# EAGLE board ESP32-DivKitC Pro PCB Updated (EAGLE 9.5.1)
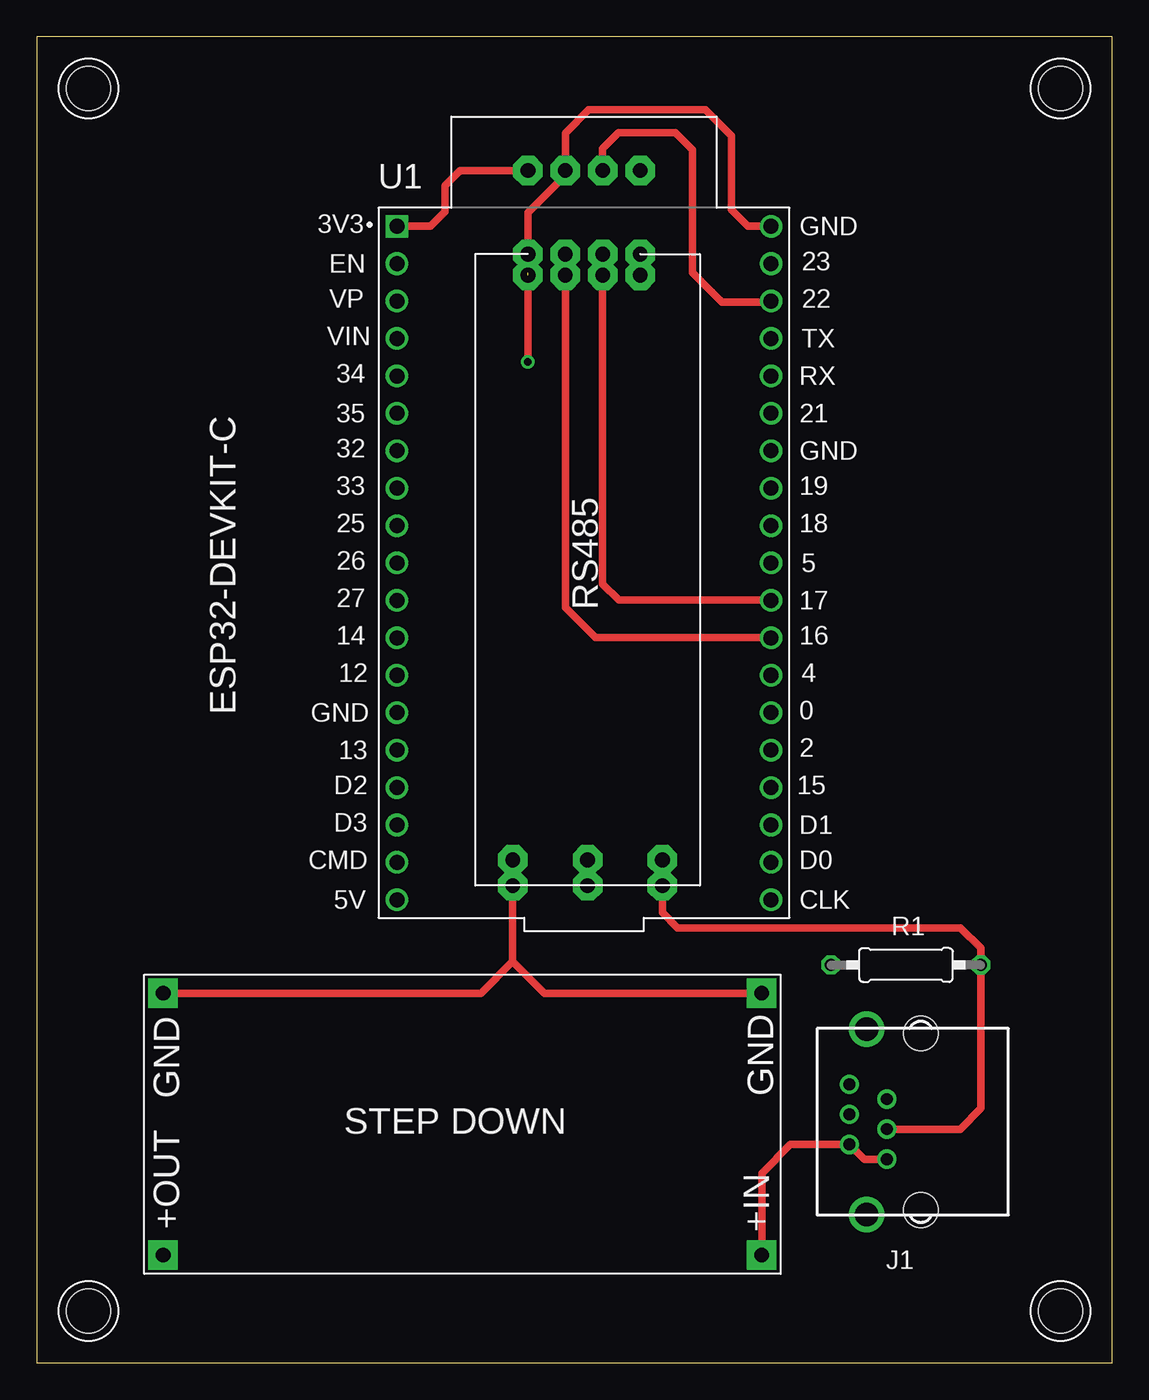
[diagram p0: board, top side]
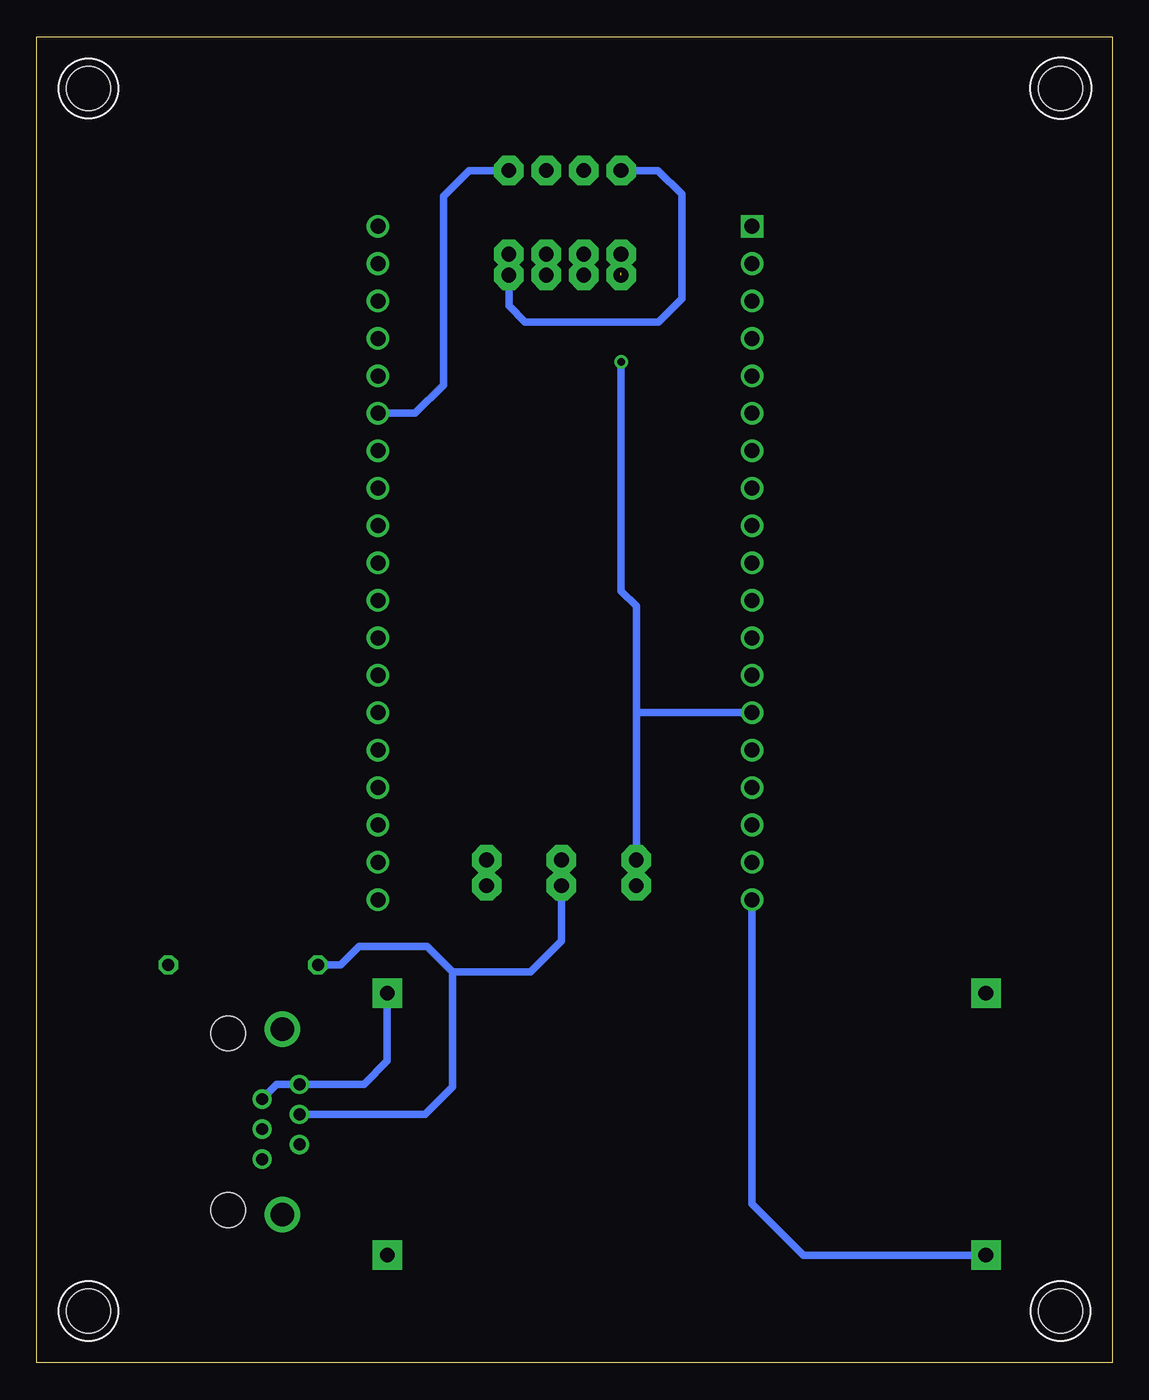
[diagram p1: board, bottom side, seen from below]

Size 73 x 90 mm. Coordinates in mm from the lower left corner, seen from the top.
Outline: 0,0 73,0 73,90 0,90 0,0
Copper layers (1*16): Top 0.035mm / dielectric 1.5mm / Bottom 0.035mm
Design rules "default *": minimum track width 6mil, minimum drill 0.2mm, track to track 6mil, track to pad 6mil, pad to pad 6mil, via to via 6mil, smd to smd 6mil, copper to edge 40mil, drill to drill 6mil, minimum pad ring 10mil, minimum via ring 8mil, stop-mask expansion 4mil, vias tented up to drill 0mil, thermal gap 10mil
Holes 3 mm at 3.5,3.5 3.5,86.5 69.5,86.5 69.5,3.5

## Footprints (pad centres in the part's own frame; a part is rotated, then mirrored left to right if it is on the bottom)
YH-55-10 = drill 0.8 pad 1.3: 1 -2.54,2.3; 2 -1.54,4.84; 3 -0.5,2.3; 4 0.5,4.84; 5 1.54,2.3; 6 2.54,4.84 | drill 1.6 pad 2.184: S1 -6.3,3.68; S2 6.3,3.68 | hole 2.36: -6,0; 6,0
0207/10 = drill 0.813 octagon: 1 -5.08,0; 2 5.08,0
MODULE_ESP32-DEVKITC = drill 1.02 square: 1 -12.7,22.85 | drill 1.02: 2 -12.7,20.31; 3 -12.7,17.77; 4 -12.7,15.23; 5 -12.7,12.69; 6 -12.7,10.15; 7 -12.7,7.61; 8 -12.7,5.07; 9 -12.7,2.53; 10 -12.7,-0.01; 11 -12.7,-2.55; 12 -12.7,-5.09; 13 -12.7,-7.63; 14 -12.7,-10.17; 15 -12.7,-12.71; 16 -12.7,-15.25; 17 -12.7,-17.79; 18 -12.7,-20.33; 19 -12.7,-22.87; 20 12.7,-22.87; 21 12.7,-20.33; 22 12.7,-17.79; 23 12.7,-15.25; 24 12.7,-12.71; 25 12.7,-10.17; 26 12.7,-7.63; 27 12.7,-5.09; 28 12.7,-2.55; 29 12.7,-0.01; 30 12.7,2.53; 31 12.7,5.07; 32 12.7,7.61; 33 12.7,10.15; 34 12.7,12.69; 35 12.7,15.23; 36 12.7,17.77; 37 12.7,20.31; 38 12.7,22.85

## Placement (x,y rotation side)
J1  RJ11  [YH-55-10]  60.01,16.35 90 top
R1  120R  [0207/10]  59,27 0 top
U1  ESP32-DEVKITC  [MODULE_ESP32-DEVKITC]  37.15,54.29 0 top

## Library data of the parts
J1 = con-wenzhou-yihua
R1 = rcl
U1 = ESP32-DEVKITC; AVAILABILITY: In Stock; DESCRIPTION: - ESP32-WROOM32 Transceiver; 802.11 b/g/n (Wi-Fi, WiFi, WLAN), Bluetooth® Smart 4.x Low Energy (BLE) 2.4GHz Evaluation Board; MF: Olimex LTD; MP: ESP32-DEVKITC; PACKAGE: None; PRICE: None; PURCHASE-URL: https://pricing.snapeda.com/search/part/ESP32-DEVKITC/?ref=eda

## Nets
3V3: U1.1
EXT_5V: U1.19
GND: J1.5 J1.6 U1.14 U1.38
GND2: U1.32
S$2: J1.1 J1.2
S$3: J1.3 R1.2
S$38: J1.4 R1.1

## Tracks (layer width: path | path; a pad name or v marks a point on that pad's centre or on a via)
3V3  (via drill 1 pad 2)
  Top 0.508: 40.96,73.98 v40.96,75.25 v40.96,73.82 | U1.1 26.72,77.14 27.7,78.12 27.7,79.88 28.74,80.92 v33.34,80.92
  Bottom 0.508: v33.34,80.92 30.82,80.92 29.21,79.31 29.21,72.23 30.8,70.64 39.85,70.64 40.96,71.75 v40.96,73.82
EXT_5V  (via drill 1 pad 2)
  Bottom 0.508: U1.19 24.45,10.79 20.95,7.3 v8.57,7.3
GND  (via drill 0.5 pad 0.7, 1 pad 2)  (1 unrouted)
  Top 0.508: 33.34,73.98 v33.34,75.25 33.34,78.06 35.88,80.61 v35.88,80.92 35.88,83.46 37.47,85.05 45.4,85.05 47.15,83.3 47.15,78.26 48.27,77.14 U1.38 | v32.31,34.13 v32.31,32.38 32.31,27.23 | v33.34,73.82 v33.34,67.94 | v49.21,25.08 34.45,25.08 32.31,27.23 | v8.57,25.08 30.16,25.08 32.31,27.23
  Bottom 0.508: v33.34,67.94 33.34,52.39 32.31,51.36 32.31,44.13 | 32.31,44.13 v32.31,34.13 | v49.21,25.08 49.21,20.48 50.8,18.89 J1.6 56.71,18.89 J1.5 | U1.14 32.3,44.12 32.31,44.13
S$1  (via drill 1 pad 2)
  Bottom 0.508: 49.85,64.45 47.31,64.45 45.4,66.36 45.4,79.18 43.66,80.92 v40.96,80.92
S$2  (via drill 1 pad 2)
  Top 0.508: v49.21,7.3 49.21,12.86 51.16,14.81 J1.2 56.17,13.81 J1.1
S$3  (via drill 1 pad 2)
  Top 0.508: v42.47,34.13 v42.47,32.38 42.47,30.56 43.5,29.53 62.71,29.53 64.08,28.15 R1.2 64.08,17.25 62.68,15.85 J1.3
S$4  (via drill 1 pad 2)
  Top 0.508: 49.85,49.21 37.94,49.21 35.88,51.28 35.88,66.36 35.88,66.52 v35.88,75.25 v35.88,73.82
S$5  (via drill 1 pad 2)
  Top 0.508: v38.42,80.92 38.42,82.42 39.5,83.5 43.34,83.5 44.5,82.34 44.5,74 46.5,72 50,72
S$6  (via drill 1 pad 2)
  Top 0.508: 49.85,51.75 39.53,51.75 38.42,52.86 38.42,64.45 38.42,64.61 v38.42,75.25 v38.42,73.82
S$38  (via drill 1 pad 2)
  Top 0.508: R1.1 53.91,27.01
  Bottom 0.508: 44.77,26.51 39.5,26.51 37.39,28.62 v37.39,32.38 v37.39,34.13 | R1.1 52.38,27 51.12,28.26 46.51,28.26 44.77,26.51 | 44.77,26.51 44.77,18.73 46.65,16.85 J1.4

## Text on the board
tPlace: 3V3 | GND | EN | 23 | VP | 22 | VIN | TX | 34 | RX | 35 | 21 | 32 | GND | 33 | 19 | 25 | 18 | 26 | 5 | 27 | RS485 | 17 | 14 | 16 | 12 | 4 | ESP32-DEVKIT-C | 0 | GND | 13 | 2 | D2 | 15 | D3 | D1 | CMD | D0 | 5V | CLK | GND | GND | STEP DOWN | +IN | +OUT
